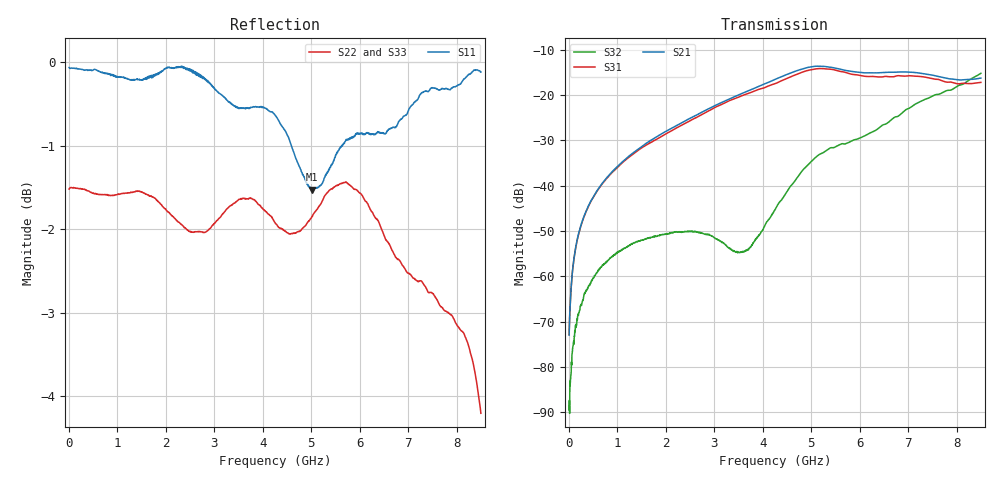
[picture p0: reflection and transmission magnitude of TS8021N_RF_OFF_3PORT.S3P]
!Agilent Technologies,E5071C,MY46522130,B.12.04
!Date: Mon Jun 30 18:15:44 2025
!Data & Calibration Information:
!Freq	S11:SOLT4(ON)	S12:SOLT4(ON)	S13:SOLT4(ON)
!	S21:SOLT4(ON)	S22:SOLT4(ON)	S23:SOLT4(ON)
!	S31:SOLT4(ON)	S32:SOLT4(ON)	S33:SOLT4(ON)
!PortZ  Port1:50+j0  Port2:50+j0  Port3:50+j0
!Above PortZ is port z conversion or system Z0 setting when saving the data.
!When reading, reference impedance value at option line is always used.
# Hz S dB R 50
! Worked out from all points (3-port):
!   1601 points, 10 MHz to 8.5 GHz, reference 50 ohm
!   strongest paths, dB at 10 MHz, 2.132 GHz, 4.255 GHz, 6.378 GHz, 8.5 GHz:
!     S21: -73.0, -27.3, -16.6, -15.1, -16.3
!     S31: -72.9, -27.8, -17.5, -16.0, -17.2
!     S32: -89.5, -50.4, -45.3, -27.5, -15.2
!   lowest |S11| = -1.5 dB at 5.014 GHz (marker M1), VSWR 11.41, Z = 4.44 + j5.74 ohm
!   |S11| at or under -10 dB: nowhere
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1e7  -0.06 -0.4  -73.10 39.9  -73.08 39.9
     -72.99 36.6  -1.52 179.8  -94.99 92.3
     -72.89 43.4  -89.51 95.9  -1.51 179.8
2.2225e8  -0.08 -10.3  -49.97 88.4  -50.11 88.1
          -49.97 88.8  -1.52 177.1  -67.66 87.0
          -50.04 87.9  -67.60 86.0  -1.51 177.8
7.900188e8  -0.13 -33.3  -38.23 92.5  -38.40 91.6
            -38.23 92.6  -1.58 168.0  -56.81 79.1
            -38.37 91.6  -56.83 79.0  -1.62 168.3
2.371281e9  -0.07 -80.1  -25.93 82.9  -26.40 82.4
            -25.92 82.9  -1.97 140.1  -50.22 48.4
            -26.44 82.2  -50.25 48.0  -1.93 141.3
3.612944e9  -0.55 -113.7  -19.49 62.6  -20.04 61.5
            -19.50 62.6  -1.63 112.6  -54.97 -58.0
            -20.01 62.2  -54.54 -57.8  -1.63 111.9
4.255e9  -0.63 -140.1  -16.59 47.7  -17.33 46.8
         -16.58 47.6  -1.92 105.3  -45.03 -125.6
         -17.51 47.4  -45.30 -122.3  -1.76 105.4
5.013794e9  -1.53 166.8  -13.79 17.3  -14.25 19.4
            -13.79 17.3  -1.85 87.5  -34.22 -165.2
            -14.42 18.8  -34.59 -166.1  -1.88 92.7
5.809731e9  -0.92 103.1  -14.79 -13.1  -15.37 -12.1
            -14.79 -13.2  -1.48 85.6  -30.30 156.5
            -15.38 -12.8  -30.32 155.5  -1.55 85.3
7.26895e9  -0.37 57.4  -15.23 -42.1  -15.97 -37.1
           -15.22 -42.1  -2.62 65.9  -21.34 121.7
           -15.94 -35.9  -21.37 122.7  -2.62 75.4
8.5e9  -0.12 60.8  -16.32 -51.0  -17.09 -43.0
       -16.28 -51.3  -4.20 42.8  -15.11 89.8
       -17.23 -44.3  -15.22 89.5  -3.93 49.8
